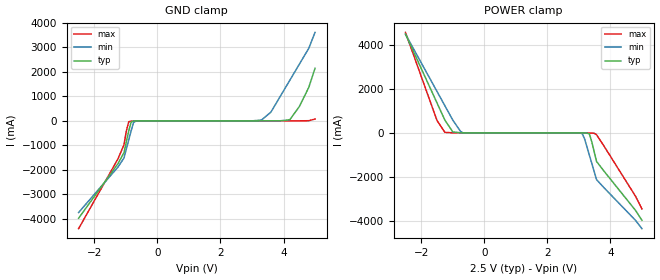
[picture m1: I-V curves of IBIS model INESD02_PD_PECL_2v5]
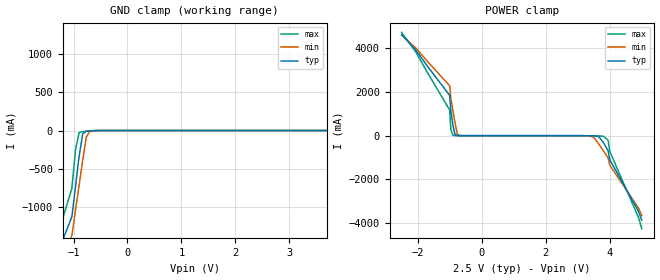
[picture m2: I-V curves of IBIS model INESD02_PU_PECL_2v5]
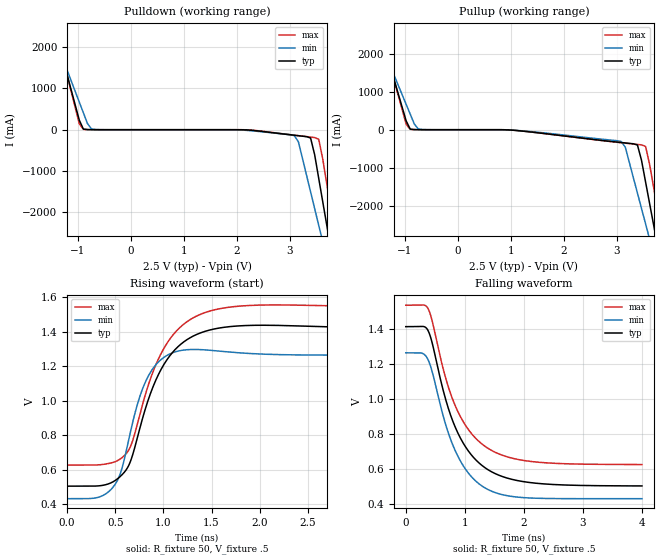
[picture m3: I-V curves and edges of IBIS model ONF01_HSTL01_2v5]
|   This file is an IBIS representation of the   |
|   Integrated Devices Technology, Inc.   |
|   ICS85310I-21   |
|LOW SKEW, DUAL, 1-TO-5 DIFFERENTIAL-TO-2.5V/3.3V ECL/LVPECL FANOUT BUFFER |
[IBIS Ver]   4.1
[File name]   85310i_21.ibs
[File Rev]   1.0
[Date]   19 Mar 2009 | Last modified
|   23 Dec 2008 | Generated
[Source]   Originated at Integrated Devices Technology, Inc.
[Disclaimer]
IDT hereby grants the user of this IBIS model a non-exclusive,
nontransferable license to use this IBIS model under the following terms.
Before using this IBIS model, the user should read this license.
If the user does not accept these terms,  the IBIS model should be
returned to IDT within 30 days.
   The user is granted this license only to use the IBIS model and
is not granted rights to sell, load, rent, lease or license the IBIS
model in whole or in part, or in modified form to anyone other than
user. User may modify the IBIS model to suit its specific
applications but rights to derivative works and such modifications
shall belong to IDT.
   This IBIS model is provided on an "AS IS" basis and IDT makes
absolutely no warranty with respect to the information contained
herein. IDT DISCLAIMS AND CUSTOMER WAIVES ALL WARRANTIES, EXPRESS
OR IMPLIED, INCLUDING WARRANTIES OF MERCHANTABILITY OR FITNESS FOR
A PARTICULAR PURPOSE. The entire risk as to quality and performance
is with the Customer. ACCORDINGLY, IN NO EVENT SHALL THE COMPANY BE
LIABLE FOR ANY DAMAGES, WHETHER IN CONTRACT OR TORT,INCLUDING ANY
LOST PROFITS OR OTHER INCIDENTAL, CONSEQUENTIAL, EXEMPLARY, OR
PUNITIVE DAMAGES ARISING OUT OF THE USE OR APPLICATION OF THE IBIS
model provided in this package. Further, IDT reserves the right to
make changes without notice to any product herein to improve
reliability, function, or design. IDT does not convey any license
under patent rights or any other intellectual property rights,
including those of third parties.
   IDT is not obligated to provide maintenance or support
for the licensed IBIS model.
[Copyright]   Copyright 2008 by Integrated Devices Technology, Inc.
[Component]   ICS85310I-21
[Manufacturer] Integrated Devices Technology, Inc.
[Package]
|LQFP32
|lead+wire  typ   min   max
R_pkg   220.4m   212.5m   238m
L_pkg   1.841n   1.708n   1.974n
C_pkg   0.316p   0.2907p   0.33p
[Pin]   signal_name   model_name   R_pin   L_pin   C_pin
1   VCC   POWER   238m   1.974n   0.330p
2   NC   NC   225m   1.841n   0.311p
3   CLKA   INESD02_PD_PECL   218m   1.7745n   0.301p
4   nCLKA   INESD02_PU_PECL   213m   1.708n   0.291p
5   NC   NC   213m   1.708n   0.291p
6   CLKB   INESD02_PD_PECL   218m   1.7745n   0.301p
7   nCLKB   INESD02_PD_PECL   225m   1.841n   0.311p
8   VEE   GND   238m   1.974n   0.330p
9   VCCO   POWER   238m   1.974n   0.330p
10   nQB4   ONF01_HSTL01   225m   1.841n   0.311p
11   QB4   ONF01_HSTL01   218m   1.7745n   0.301p
12   nQB3   ONF01_HSTL01   213m   1.708n   0.291p
13   QB3   ONF01_HSTL01   213m   1.708n   0.291p
14   nQB2   ONF01_HSTL01   218m   1.7745n   0.301p
15   QB2   ONF01_HSTL01   225m   1.841n   0.311p
16   VCCO   POWER   238m   1.974n   0.330p
17   nQB1   ONF01_HSTL01   238m   1.974n   0.330p
18   QB1   ONF01_HSTL01   225m   1.841n   0.311p
19   nQB0   ONF01_HSTL01   218m   1.7745n   0.301p
20   QB0   ONF01_HSTL01   213m   1.708n   0.291p
21   nQA4   ONF01_HSTL01   213m   1.708n   0.291p
22   QA4   ONF01_HSTL01   218m   1.7745n   0.301p
23   nQA3   ONF01_HSTL01   225m   1.841n   0.311p
24   QA3   ONF01_HSTL01   238m   1.974n   0.330p
25   VCCO   POWER   238m   1.974n   0.330p
26   nQA2   ONF01_HSTL01   225m   1.841n   0.311p
27   QA2   ONF01_HSTL01   218m   1.7745n   0.301p
28   nQA1   ONF01_HSTL01   213m   1.708n   0.291p
29   QA1   ONF01_HSTL01   213m   1.708n   0.291p
30   nQA0   ONF01_HSTL01   218m   1.7745n   0.301p
31   QA0   ONF01_HSTL01   225m   1.841n   0.311p
32   VCC0   POWER   238m   1.974n   0.330p
[Diff Pin] inv_pin  vdiff tdelay_typ tdelay_min  tdelay_max
|Output
11   10   NA   0   0   0
13   12   NA   0   0   0
15   14   NA   0   0   0
18   17   NA   0   0   0
20   19   NA   0   0   0
22   21   NA   0   0   0
24   23   NA   0   0   0
27   26   NA   0   0   0
29   28   NA   0   0   0
31   30   NA   0   0   0
|Input
3   4   .15   0   0   0
6   7   .15   0   0   0
[Model Selector] INESD02_PD_PECL
INESD02_PD_PECL_2v5  Buffer selection for 2v5
INESD02_PD_PECL_3v3  Buffer selection for 3v3
[Model Selector] INESD02_PU_PECL
INESD02_PU_PECL_2v5  Buffer selection for 2v5
INESD02_PU_PECL_3v3  Buffer selection for 3v3
[Model Selector] ONF01_HSTL01
ONF01_HSTL01_2v5  Buffer selection for 2v5
ONF01_HSTL01_3v3  Buffer selection for 3v3
| Models and submodels in the file (6): INESD02_PD_PECL_2v5 (Input), INESD02_PU_PECL_2v5 (Input), ONF01_HSTL01_2v5 (Output_ECL), INESD02_PD_PECL_3v3 (Input), INESD02_PU_PECL_3v3 (Input), ONF01_HSTL01_3v3 (Output_ECL)
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[Model] INESD02_PD_PECL_2v5
Model_type   Input
Polarity   Non-Inverting
Vinl = 0.8V
Vinh = 2.0V
|   typ   min   max
C_comp   2pF   1.5pF   2.5pF
|   typ   min   max
[Voltage range]  2.5V   2.375V   2.625V
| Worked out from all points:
|   GND clamp passes 1 mA (typ) near -0.59 V on its own axis
|   POWER clamp passes 1 mA (typ) near -0.69 V on its own axis
[GND_clamp]
|Voltage   I(typ)   I(min)   I(max)
-2.5V     -3.983A    -3.749A    -4.408A
-1.25V    -1.747A    -1.889A    -1.551A
-1.061V   -1.3A      -1.517A    -979.1mA
-909.1mV  -407.1mA   -774.3mA   -35.24mA
-833.3mV  -48.47mA   -403.4mA   -14.47mA
-757.6mV  -7.272mA   -70.21mA   -9.677mA
-681.8mV  -2.863mA   -7.067mA   -5.73mA
3.3V      167.2uA    32.81mA    49.66uA
3.6V      586.4uA    357.8mA    70.1uA
4.2V      47.81mA    1.661A     649.6uA
4.8V      1.366A     2.965A     5.596mA
5V        2.15A      3.618A     75.79mA
[POWER_clamp]
|Voltage   I(typ)   I(min)   I(max)
-2.5V     4.503A     4.499A     4.579A
-1.5V     1.366A     1.889A     566.5mA
-1.25V    582.4mA    1.237A     24.21mA
-1V       47.81mA    585.7mA    3.595mA
-681.8mV  586.4uA    6.896mA    416.8uA
3.03V     -323.1uA   -3.378mA   -47.98uA
3.106V    -1.127mA   -30.71mA   -286.5uA
3.182V    -2.863mA   -273.7mA   -1.276mA
3.333V    -48.47mA   -1.016A    -7.036mA
3.561V    -1.3A      -2.13A     -81.94mA
4.8V      -3.536A    -3.991A    -2.894A
5V        -3.983A    -4.363A    -3.465A
[Model] INESD02_PU_PECL_2v5
Model_type   Input
Polarity   Non-Inverting
Vinl = .8V
Vinh =  2V
|   typ   min   max
C_comp   2pF   1.5pF   2.5pF
|   typ   min   max
[Voltage range]  2.5V   2.375V   2.625V
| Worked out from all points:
|   GND clamp passes 1 mA (typ) near -0.59 V on its own axis
|   POWER clamp passes 1 mA (typ) near -0.70 V on its own axis
[GND_clamp]
|Voltage   I(typ)   I(min)   I(max)
-2.5V     -3.894A    -3.674A    -4.294A
-1.25V    -1.521A    -1.7A      -1.261A
-1.031V   -1.125A    -1.372A    -755.3mA
-896.9mV  -335.4mA   -714.7mA   -27.06mA
-695.9mV  -3.401mA   -10.7mA    -6.467mA
3.995V    711.6uA    10.32mA    481.3uA
4.062V    4.029mA    88.04mA    1.401mA
4.129V    40.44mA    547.3mA    3.341mA
4.196V    445.8mA    1.124A     14.79mA
4.263V    1.139A     1.7A       275.9mA
4.5V      1.832A     2.277A     1.163A
5V        3.219A     3.431A     2.937A
[POWER_clamp]
|Voltage   I(typ)   I(min)   I(max)
-2.5V     4.617A     4.594A     4.726A
-1V       1.842A     2.286A     1.176A
-963.9mV  1.149A     1.709A     289.6mA
-896.9mV  456.4mA    1.132A     15.33mA
-829.9mV  42.02mA    556.1mA    3.389mA
-762.9mV  4.159mA    91.01mA    1.421mA
-695.9mV  727.9uA    10.67mA    490.4uA
3.35V     -3.204mA   -9.193mA   -6.2mA
3.8V      -305mA     -689.5mA   -24.7mA
3.95V     -699.9mA   -1.018A    -211mA
4V        -1.095A    -1.346A    -716.4mA
5V        -3.863A    -3.649A    -4.255A
[Model] ONF01_HSTL01_2v5
Model_type  Output_ECL
Polarity   Non-Inverting
Vmeas = .89
Rref = 50
Cref = 0
Vref = .5
|Variable  typ   min   max
C_comp   2p   1.5p   2.5p
[Voltage Range]   2.5   2.375   2.625
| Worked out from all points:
|   rising waveform, R_fixture 50, V_fixture .5: 20-80 % time 350ps typ, 240ps min, 362ps max; typ from 0.504 V to 1.42 V
|   falling waveform, R_fixture 50, V_fixture .5: 20-80 % time 591ps typ, 523ps min, 591ps max; typ from 1.41 V to 0.504 V
| Open source, no load
|  Voltage   I(typ)   I(min)   I(max)
[Pullup]
-2.5V     7.585A     5.853A     7.966A
-1.582V   3.168A     2.738A     3.268A
-1.505V   2.8A       2.478A     2.877A
-892.9mV  15.1mA     409.7mA    8.262mA
-739.8mV  1.385mA    17.35mA    1.003mA
3.087V    -338.1mA   -312.6mA   -343.9mA
3.393V    -404.5mA   -1.675A    -388.5mA
3.469V    -807.4mA   -2.079A    -400mA
3.546V    -1.379A    -2.483A    -441.2mA
3.699V    -2.523A    -3.292A    -1.528A
3.852V    -3.666A    -4.1A      -2.744A
5V        -12.24A    -10.16A    -11.86A
[Pulldown]
-2.5V     7.585A     5.853A     7.966A
-1.505V   2.8A       2.478A     2.877A
-1.429V   2.433A     2.219A     2.485A
-892.9mV  15.1mA     409.7mA    8.262mA
-663.3mV  413.9uA    3.764mA    253.1uA
3.087V    -134.5mA   -144.5mA   -132.9mA
3.393V    -201.7mA   -1.506A    -178.4mA
3.469V    -604.8mA   -1.91A     -190.2mA
3.546V    -1.177A    -2.315A    -231.7mA
3.699V    -2.321A    -3.123A    -1.319A
3.852V    -3.464A    -3.931A    -2.535A
5V        -12.04A    -9.99A     -11.65A
[Ramp]
|   typ   min   max
dV/dt_r   0.747/0.607n   0.692/0.422n   0.743/0.611n
dV/dt_f   0.728/0.954n   0.666/0.82n   0.729/0.951n
R_load =   50.0000
[Rising Waveform]
R_fixture = 50
V_fixture = .5   | VCC_typ - 2V
V_fixture_max = 0.625   | VCC_max - 2V
V_fixture_min = 0.375   | VCC_min - 2V
C_fixture = 0.0p
| Time   typ   min   max
0s        503.5mV    430.9mV    625.7mV
426.4ps   516.2mV    469mV      634.6mV
537.1ps   552.3mV    553.7mV    655.9mV
615ps     599.4mV    709mV      693.2mV
725.7ps   775.8mV    969.5mV    854.9mV
824.1ps   972.5mV    1.121V     1.055V
1.099ns   1.282V     1.278V     1.38V
1.365ns   1.389V     1.296V     1.496V
1.755ns   1.433V     1.279V     1.547V
3.997ns   1.415V     1.264V     1.538V
[Falling Waveform]
R_fixture = 50
V_fixture = .5   | VCC_typ - 2V
V_fixture_max = 0.625   | VCC_max - 2V
V_fixture_min = 0.375   | VCC_min - 2V
C_fixture = 0.0p
| Time   typ   min   max
0s        1.413V     1.264V     1.536V
270.6ps   1.415V     1.262V     1.537V
373.1ps   1.394V     1.228V     1.519V
446.9ps   1.321V     1.157V     1.446V
668.3ps   1.006V     861.8mV    1.129V
832.3ps   843.5mV    708.9mV    965.8mV
1.074ns   696.6mV    571.2mV    819.3mV
1.365ns   602.2mV    488mV      724.4mV
2.148ns   521.3mV    434.3mV    642.4mV
3.997ns   503.9mV    431mV      626mV
